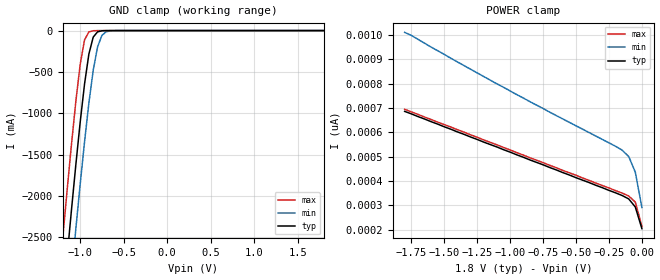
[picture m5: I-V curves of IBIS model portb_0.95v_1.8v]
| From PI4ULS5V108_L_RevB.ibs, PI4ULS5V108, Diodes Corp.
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|   Model IO_B
[Model]   portb_0.95v_1.8v
Model_type Terminator
| variable   typ   min   max
C_comp   3.5561p   3.5280p   3.5829p
[Voltage Range]   1.8000V   1.6200V   1.9800V
[POWER Clamp Reference]   1.8000V   1.6200V   1.9800V
[GND Clamp Reference]   0.0000V   0.0000V   0.0000V
[Temperature Range]   25   85   -40
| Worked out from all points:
|   GND clamp passes 1 mA (typ) near -0.71 V on its own axis
[GND Clamp]
| Voltage   I(typ)   I(min)   I(max)
-1.8V     -10.33A    -11A       -9.655A
-1.2V     -3.313A    -4.105A    -2.505A
-1.15V    -2.735A    -3.53A     -1.931A
-1.1V     -2.17A     -2.959A    -1.377A
-1.05V    -1.624A    -2.401A    -858.9mA
-1V       -1.11A     -1.861A    -410.8mA
-950mV    -647.9mA   -1.348A    -112.9mA
-900mV    -283.7mA   -877.9mA   -15.94mA
-850mV    -78.75mA   -479.3mA   -1.974mA
-800mV    -15.25mA   -197mA     -233.3uA
-700mV    -522.2uA   -13.76mA   -2.027uA
1.8V      96.53pA    125.3pA    96.01pA
[POWER Clamp]
| Voltage   I(typ)   I(min)   I(max)
-1.8V     686pA      1.01nA     695pA
-1.75V    676pA      998pA      684pA
-1.45V    613pA      904pA      622pA
-950mV    508pA      755pA      517pA
-150mV    341pA      527pA      351pA
-100mV    327pA      501pA      339pA
-50mV     294pA      437pA      314pA
0V        205pA      292pA      215pA
